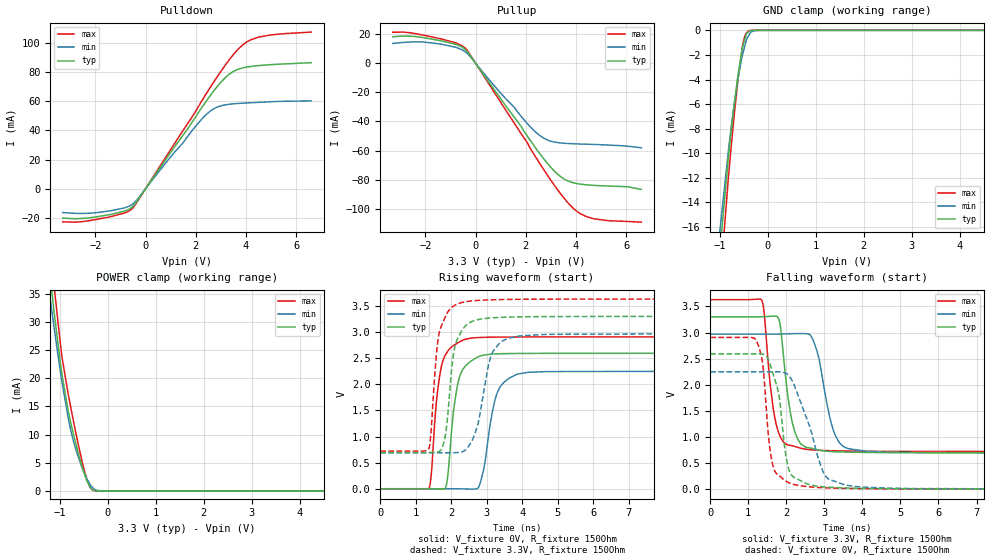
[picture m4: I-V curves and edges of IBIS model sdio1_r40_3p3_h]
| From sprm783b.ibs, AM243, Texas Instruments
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|   r40_3p3_h
[Model]   sdio1_r40_3p3_h
Model_type   I/O
Polarity   Non-Inverting
Enable   Active-High
Vinl = 0
Vinh = 0.8
Vmeas = 1.65
Vref = 3.3
Cref = 2pF
Rref = 100000
|   typ   min   max
C_comp   5.631pF   5.516pF   5.647pF
[Voltage Range]   3.3   2.97   3.63
[Temperature Range]   27   150   -40
[Pullup Reference]   3.3   2.97   3.63
[Pulldown Reference]   0   0   0
[Power Clamp Reference]   3.3   2.97   3.63
[GND Clamp Reference]   0   0   0
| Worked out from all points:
|   slope of the pulldown table from 0 to 0.495 V, typ, clamps not added: 39.9 ohm
|   slope of the pullup table from 0 to 0.495 V, typ, clamps not added: 40.8 ohm
|   GND clamp passes 1 mA (typ) near -0.50 V on its own axis
|   POWER clamp passes 1 mA (typ) near -0.39 V on its own axis
|   falling waveform, V_fixture 3.3V, R_fixture 150Ohm: 20-80 % time 284ps typ, 374ps min, 260ps max; typ from 3.3 V to 0.694 V
|   rising waveform, V_fixture 0V, R_fixture 150Ohm: 20-80 % time 267ps typ, 339ps min, 247ps max; typ from 0 V to 2.59 V
|   rising waveform, V_fixture 3.3V, R_fixture 150Ohm: 20-80 % time 252ps typ, 399ps min, 234ps max; typ from 0.694 V to 3.3 V
|   falling waveform, V_fixture 0V, R_fixture 150Ohm: 20-80 % time 309ps typ, 599ps min, 219ps max; typ from 2.59 V to 0 V
[Pulldown]
|   Voltage   I(typ)   I(min)   I(max)
-3.3V     -20.24mA   -16.35mA   -22.74mA
-2.627V   -20.51mA   -16.96mA   -22.78mA
-1.904V   -19.15mA   -16.31mA   -20.92mA
-825mV    -15.32mA   -13.09mA   -16.58mA
-528mV    -12.6mA    -10.73mA   -13.68mA
2.363V    58.81mA    50.06mA    63.75mA
2.779V    68.52mA    55.45mA    74.91mA
3.194V    76.56mA    57.64mA    85.33mA
3.472V    80.24mA    58.25mA    91.59mA
3.927V    83.16mA    58.8mA     99.52mA
4.491V    84.51mA    59.27mA    104mA
6.6V      86.52mA    60.3mA     107.5mA
[GND Clamp]
|   Voltage   I(typ)   I(min)   I(max)
-3.3V     -160mA     -119.4mA   -217mA
-1.033V   -19.39mA   -17.52mA   -22.42mA
-825mV    -10.43mA   -9.877mA   -12.11mA
-716.1mV  -6.541mA   -6.437mA   -7.501mA
-636.9mV  -4.054mA   -4.313mA   -4.508mA
-537.9mV  -1.566mA   -2.15mA    -1.56mA
-508.2mV  -1.102mA   -1.701mA   -874.9uA
-468.6mV  -579.2uA   -1.102mA   -331.5uA
-399.3mV  -111.6uA   -431.1uA   -25.79uA
-349.8mV  -18.86uA   -131.8uA   -5.146uA
-171.6mV  -88.3nA    -2.804uA   -107.4nA
6.6V      0A         0A         0A
[Pullup]
|   Voltage   I(typ)   I(min)   I(max)
-3.3V     18.22mA    13.61mA    21.27mA
-2.458V   18.42mA    14.67mA    20.52mA
-1.429V   15.6mA     13.29mA    16.94mA
-825mV    13.14mA    11.11mA    14.22mA
-409.2mV  9.448mA    7.817mA    10.39mA
2.501V    -60.79mA   -48.88mA   -67.37mA
2.858V    -68.68mA   -52.68mA   -76.8mA
3.333V    -77.15mA   -54.66mA   -88.46mA
3.887V    -82.07mA   -55.31mA   -99.54mA
4.155V    -82.98mA   -55.48mA   -103.2mA
4.729V    -83.92mA   -55.76mA   -106.9mA
6.6V      -86.67mA   -58.06mA   -109.2mA
[POWER Clamp]
|   Voltage   I(typ)   I(min)   I(max)
-3.3V     224.5mA    191.3mA    262.6mA
-1.211V   38.57mA    34.7mA     44.22mA
-1.132V   32.63mA    29.7mA     37.31mA
-1.122V   31.9mA     29.08mA    36.46mA
-953.7mV  20.54mA    19.22mA    23.62mA
-825mV    14.09mA    12.89mA    17.14mA
-765.6mV  11.78mA    10.49mA    14.49mA
-636.9mV  7.357mA    6.549mA    9.056mA
-468.6mV  2.565mA    2.754mA    2.952mA
-399.3mV  1.162mA    1.587mA    1.169mA
-290.4mV  108.4uA    386uA      43.42uA
6.6V      0A         0A         0A
[Ramp]
R_load = 150
|   typ   min   max
dV/dt_r   1.55545/2.66804e-10   1.3484/3.38592e-10   1.74402/2.46044e-10
dV/dt_f   1.56311/2.81324e-10   1.36817/3.74112e-10   1.74583/2.59491e-10
[Falling Waveform]
V_fixture = 3.3V
V_fixture_min = 2.97V
V_fixture_max = 3.63V
R_fixture = 150Ohm
C_fixture = 0F
|   Time   V(typ)   V(min)   V(max)
0s        3.3V       2.969V     3.63V
1.355ns   3.302V     2.969V     3.622V
1.59ns    3.312V     2.97V      1.915V
1.79ns    3.277V     2.971V     1.099V
2.03ns    1.832V     2.975V     849.7mV
2.3ns     957.7mV    2.98V      799.9mV
2.675ns   779.8mV    2.9V       752.4mV
3.225ns   719mV      1.152V     735.9mV
3.595ns   709.7mV    784.6mV    731.3mV
10ns      694.5mV    689mV      720mV
[Rising Waveform]
V_fixture = 0V
V_fixture_min = 0V
V_fixture_max = 0V
R_fixture = 150Ohm
C_fixture = 0F
|   Time   V(typ)   V(min)   V(max)
0s        414.8uV    957.9uV    279.3uV
1.38ns    231.3uV    629.3uV    10.69mV
1.615ns   -2.694mV   458.4uV    1.862V
1.83ns    1.683mV    493.2uV    2.553V
2.1ns     1.66V      -393.4uV   2.757V
2.335ns   2.291V     -2.229mV   2.846V
2.785ns   2.532V     46.6mV     2.894V
3.285ns   2.582V     1.817V     2.901V
3.855ns   2.588V     2.192V     2.904V
10ns      2.593V     2.248V     2.907V
[Rising Waveform]
V_fixture = 3.3V
V_fixture_min = 2.97V
V_fixture_max = 3.63V
R_fixture = 150Ohm
C_fixture = 0F
|   Time   V(typ)   V(min)   V(max)
0s        694.5mV    689mV      720mV
1.37ns    694.3mV    688.8mV    766.3mV
1.655ns   711.6mV    688.7mV    2.963V
1.83ns    995.3mV    688.7mV    3.285V
2.03ns    2.396V     688.8mV    3.479V
2.165ns   2.853V     692mV      3.533V
2.61ns    3.207V     954.1mV    3.596V
3.13ns    3.27V      2.559V     3.616V
3.605ns   3.284V     2.879V     3.623V
10ns      3.3V       2.969V     3.63V
[Falling Waveform]
|Gnd
V_fixture = 0V
V_fixture_min = 0V
V_fixture_max = 0V
R_fixture = 150Ohm
C_fixture = 0F
|   Time   V(typ)   V(min)   V(max)
0s        2.593V     2.248V     2.907V
1.21ns    2.593V     2.248V     2.854V
1.38ns    2.588V     2.248V     2.386V
1.53ns    2.474V     2.248V     1.017V
1.64ns    2.233V     2.248V     472.8mV
1.8ns     1.829V     2.248V     265.6mV
1.965ns   754.5mV    2.228V     166.2mV
2.095ns   321.3mV    2.145V     114.8mV
3.12ns    37.93mV    189.8mV    23.51mV
10ns      412.9uV    958uV      279.6uV
